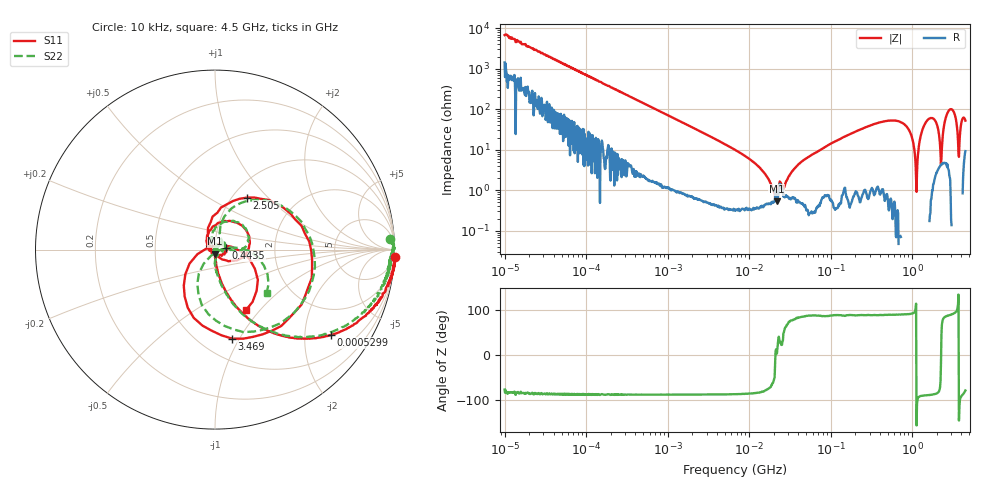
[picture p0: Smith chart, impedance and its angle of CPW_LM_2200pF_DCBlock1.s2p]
!Siglent Technologies,SNA5004A,SNA5XCED5R0097,V1.0.0.2.10.R9
!Date: 2024-10-28 16:34:14
!Data & Calibration Information:
!Freq	S11:F2(ON)	S21:F2(ON)	S12:F2(ON)	S22:F2(ON)
# Hz S DB R 50
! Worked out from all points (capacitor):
!   1001 points, 10 kHz to 4.5 GHz, reference 50 ohm
!   read as one part in series: C = 2.28 nF near 10.67 kHz
!   lowest |Z| = 533 mohm at 21.93 MHz (marker M1)
!   series resonance near 20.99 MHz, so ESL is about 25 nH
!   S11 on the Smith chart (normalised r, x): 10 kHz: -7, -48; 529.9 kHz: 1.01, -2.71; 443.5 MHz: 1.13, +0.02; 2.505 GHz: 1.17, +0.76; 3.469 GHz: 0.70, -0.93; 4.5 GHz: 1.07, -0.85
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10000  0.05 -2.3  -36.73 78.4  -37.38 80.6  -0.21 3.5
87919.76  -0.01 -7.1  -18.30 82.4  -18.29 82.4  -0.26 -6.9
529943.8  -1.91 -36.4  -4.61 52.8  -4.60 52.8  -2.14 -36.6
772988.4  -3.36 -46.9  -2.79 42.3  -2.80 42.4  -3.59 -47.1
6708204  -19.57 -84.4  -0.13 5.2  -0.12 5.1  -19.13 -87.9
2.19305e7  -32.86 -88.9  -0.07 -1.7  -0.05 -1.6  -29.04 -79.5
4.315346e7  -42.41 -76.2  -0.06 -5.8  -0.06 -5.8  -48.19 30.2
5.897837e7  -47.36 31.6  -0.09 -8.5  -0.07 -8.5  -39.97 160.9
7.26347e7  -40.33 69.0  -0.08 -10.8  -0.06 -10.8  -57.38 -94.2
1.005714e8  -38.65 65.3  -0.10 -15.3  -0.05 -15.2  -31.65 66.9
4.435481e8  -24.45 7.8  -0.22 -68.2  -0.16 -67.9  -23.80 14.1
5.185364e8  -24.60 -5.8  -0.20 -79.7  -0.16 -79.4  -24.45 16.6
6.995248e8  -28.05 -51.3  -0.23 -107.4  -0.16 -107.1  -29.82 -1.6
8.177898e8  -32.31 -116.0  -0.24 -125.6  -0.19 -125.3  -42.27 47.9
1.132327e9  -19.30 107.1  -0.30 -174.4  -0.27 -174.0  -19.54 94.8
1.717413e9  -14.46 2.8  -0.54 96.1  -0.51 96.6  -14.44 15.5
2.087723e9  -32.64 -96.2  -0.46 37.4  -0.45 37.9  -24.62 24.8
2.505059e9  -9.36 58.3  -1.28 -30.8  -1.26 -30.1  -9.23 52.8
2.928576e9  -5.29 -6.1  -2.61 -91.2  -2.57 -90.5  -5.20 -0.7
3.468552e9  -5.92 -79.1  -2.45 -162.5  -2.43 -161.5  -5.94 -64.7
4.002521e9  -27.91 163.9  -0.98 113.1  -1.01 112.4  -27.63 -123.2
4.5e9  -8.43 -62.9  -1.84 30.5  -1.92 29.7  -8.47 -40.3
